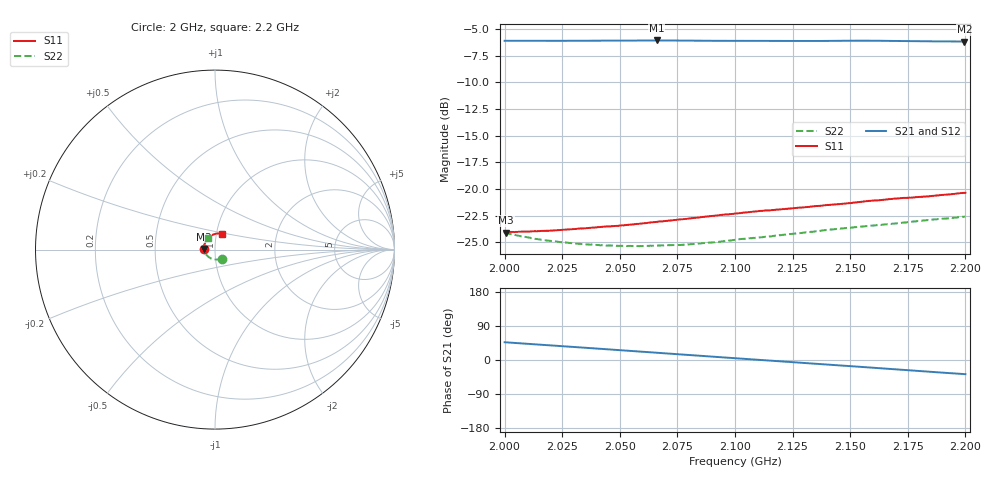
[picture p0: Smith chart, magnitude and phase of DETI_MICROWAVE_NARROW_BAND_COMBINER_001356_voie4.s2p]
! 12/28/2020 4:23:00 PM
! \\DETI-AD\SERVEUR COMMUN\0\01 - PRODUIT\0 01 356 - COMBINEUR 4 VOIES BANDE S 800 WATTS\81 -PROCES VERBAL DE CONTROLE\MESURES\07 - S2P\VOIE4.S2P
! CHANNEL.1
! TR.MEASUREMENT
! CORRECTED.DATA
# GHZ S RI R 50.0
! FREQ.GHZ  S11RE  S11IM  S21RE  S21IM  S12RE  S12IM  S22RE  S22IM
!; PortSelection: Port_12
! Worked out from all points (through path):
!   1000 points, 2 GHz to 2.2 GHz, reference 50 ohm
!   highest |S21| = -6.08 dB at 2.066 GHz (marker M1); lowest = -6.2 dB at 2.2 GHz (marker M2)
!   lowest |S11| = -24.1 dB at 2.001 GHz (marker M3), VSWR 1.13, Z = 44.1 + j0.293 ohm
!   |S11| at or under -10 dB: start of sweep to end of sweep
!   |S22| runs from -25.4 to -22.6 dB; largest |S21 - S12| = 0.0022
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2  -0.0626 0.00285  0.3382 0.361  0.3382 0.3614  0.0373 -0.05
2.000601  -0.0624 0.00331  0.34 0.3594  0.3396 0.36  0.0366 -0.0503
2.006406  -0.0626 0.0075  0.3547 0.3447  0.3549 0.3451  0.0301 -0.0522
2.015616  -0.0619 0.0144  0.3766 0.3202  0.377 0.3204  0.0198 -0.0544
2.024825  -0.0608 0.0209  0.3974 0.2943  0.3979 0.2944  0.00946 -0.0555
2.033433  -0.0594 0.0269  0.4153 0.2691  0.4158 0.2689  0.000191 -0.0552
2.049249  -0.0558 0.0374  0.4444 0.2196  0.4446 0.2188  -0.0162 -0.0517
2.059459  -0.0528 0.0442  0.4603 0.1854  0.4601 0.1849  -0.0258 -0.0475
2.066066  -0.0507 0.0485  0.469 0.1628  0.4684 0.162  -0.0317 -0.0441
2.066667  -0.0507 0.0489  0.4697 0.1605  0.4691 0.1599  -0.0322 -0.0438
2.076076  -0.047 0.0546  0.4794 0.1273  0.4788 0.1271  -0.0394 -0.0379
2.080681  -0.0451 0.0573  0.4829 0.1109  0.4826 0.1108  -0.0428 -0.0348
2.092893  -0.0397 0.0641  0.4898 0.0665  0.4897 0.0667  -0.0505 -0.0255
2.1001  -0.0359 0.0678  0.4924 0.0404  0.4925 0.0405  -0.0544 -0.0196
2.115716  -0.0273 0.0748  0.4936 -0.0146  0.4939 -0.015  -0.0597 -0.00592
2.133534  -0.0162 0.0812  0.4874 -0.0783  0.4867 -0.0796  -0.0622 0.0103
2.140541  -0.0112 0.0834  0.483 -0.1039  0.4819 -0.1049  -0.0622 0.0167
2.150751  -0.00367 0.0859  0.4746 -0.1408  0.4729 -0.1411  -0.0606 0.026
2.166767  0.00843 0.0892  0.4537 -0.1955  0.452 -0.1946  -0.0554 0.0402
2.186987  0.0252 0.0896  0.4163 -0.2609  0.4164 -0.2599  -0.0454 0.0561
2.1996  0.036 0.0889  0.3908 -0.297  0.3908 -0.2965  -0.037 0.0643
2.2  0.0363 0.0889  0.3899 -0.2982  0.3901 -0.2977  -0.0366 0.0646
